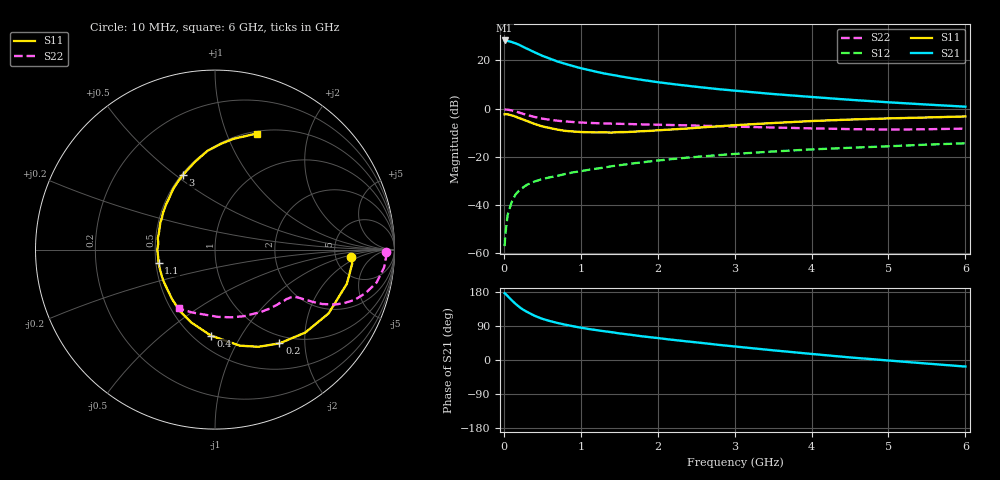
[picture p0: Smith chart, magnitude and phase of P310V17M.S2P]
! SIEMENS Small Signal Semiconductors
! BFP181
! Si NPN RF Bipolar Junction Transistor in SOT143
! VCE = 10 V  IC = 17 mA
! Common Emitter S-Parameters:  March  1996
# GHz  S  MA  R  50
!  f  S11  S21  S12  S22
! GHz  MAG  ANG  MAG  ANG  MAG  ANG  MAG  ANG
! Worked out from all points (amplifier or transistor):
!   36 points, 10 MHz to 6 GHz, reference 50 ohm
!   highest |S21| = 28.3 dB at 10 MHz (marker M1)
!   |S21| within 3 dB of that: start of sweep to 273.8 MHz
!   unconditionally stable (mu >= 1): 1.075 GHz to end of sweep
!   at 250 MHz: K = 0.42, MSG = 29.2 dB, |S12| = -32.7 dB
!   at 1.4 GHz: K = 1.08, MAG = 17.2 dB, |S12| = -23.9 dB
!   at 6 GHz: K = 1.02, MAG = 6.7 dB, |S12| = -14.4 dB
!   S11 on the Smith chart (normalised r, x): 10 MHz: 7.13, -1.31; 200 MHz: 0.87, -1.53; 400 MHz: 0.60, -0.75; 1.1 GHz: 0.52, -0.09; 3 GHz: 0.51, +0.53; 6 GHz: 0.52, +1.28
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0.01  0.7612 -2.9  25.88 176.1  0.0014 59.0  0.9553 -0.8
0.02  0.7683 -5.9  25.61 174.9  0.0025 72.0  0.955 -2.1
0.05  0.759 -14.5  25.29 168.6  0.0063 81.3  0.9478 -5.9
0.1  0.7261 -29.3  24.12 158.2  0.0113 70.3  0.919 -11.5
0.15  0.683 -42.6  22.59 148.6  0.0164 67.9  0.8744 -16.0
0.2  0.634 -55.5  20.97 140.1  0.0201 63.6  0.827 -19.8
0.25  0.5932 -65.9  19.09 132.8  0.0231 60.4  0.7789 -22.5
0.3  0.5528 -75.5  17.52 127.2  0.0263 58.1  0.7376 -24.5
0.4  0.4793 -92.8  14.72 116.6  0.0308 55.1  0.6704 -26.9
0.5  0.427 -108.0  12.45 108.7  0.0345 53.0  0.6194 -28.1
0.6  0.3949 -119.6  10.85 102.7  0.0376 52.9  0.5841 -28.8
0.7  0.3655 -130.7  9.443 97.6  0.0404 52.7  0.559 -29.4
0.9  0.3353 -149.8  7.614 89.1  0.0476 52.1  0.5264 -30.3
1.1  0.3232 -166.5  6.332 81.9  0.0536 52.8  0.5054 -31.5
1.3  0.3214 -179.9  5.371 76.0  0.0597 52.3  0.493 -33.3
1.6  0.326 163.6  4.42 67.8  0.0701 51.3  0.4793 -36.3
2.2  0.3703 137.5  3.219 53.1  0.0901 48.0  0.4551 -44.3
3  0.4516 113.6  2.358 35.7  0.1147 42.0  0.4224 -56.9
3.5  0.5014 102.9  2.005 25.6  0.1288 38.0  0.4052 -66.2
4.5  0.5918 86.5  1.522 6.8  0.1539 29.6  0.3752 -87.5
5.5  0.654 75.1  1.212 -9.4  0.1788 22.2  0.3728 -109.9
6  0.6874 70.2  1.095 -17.3  0.1907 18.3  0.3846 -121.5
